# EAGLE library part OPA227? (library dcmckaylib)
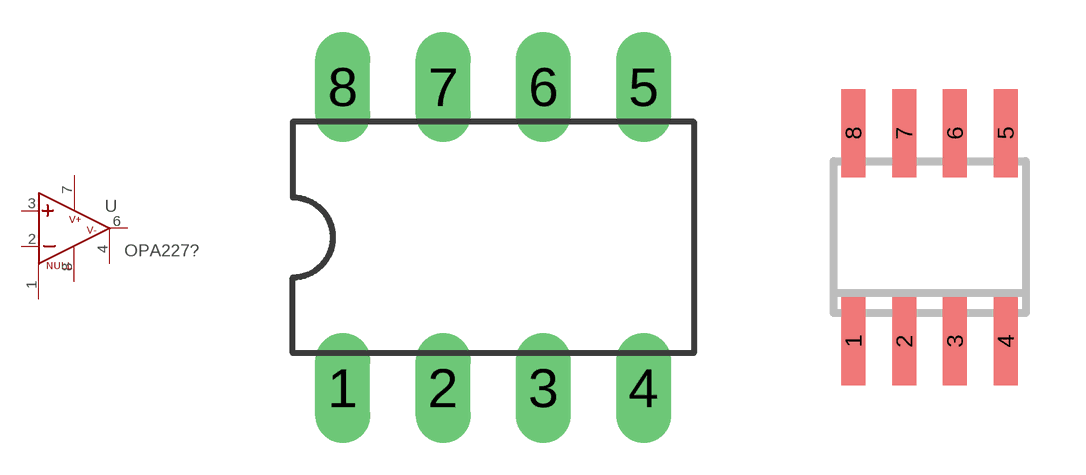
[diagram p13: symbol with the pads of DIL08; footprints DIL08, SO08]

Designator prefix U

## OPA227P  [DIL08]
1  NULL1
2  IN-  in
3  IN+  in
4  V-  pwr
6  OUT  out
7  V+  pwr
8  NULL2

## OPA227U  [SO08]
Pads as for DIL08

## Footprint DIL08 (pad centres in mm)
Dual In Line Package
drill 0.889 long: 1 -3.81,-3.81; 2 -1.27,-3.81; 3 1.27,-3.81; 4 3.81,-3.81; 5 3.81,3.81; 6 1.27,3.81; 7 -1.27,3.81; 8 -3.81,3.81

## Footprint SO08 (pad centres in mm)
Small Outline Package 8 NS Package M08A
smd 0.6 x 2.2: 1 -1.905,-2.6; 2 -0.635,-2.6; 3 0.635,-2.6; 4 1.905,-2.6; 5 1.905,2.6; 6 0.635,2.6; 7 -0.635,2.6; 8 -1.905,2.6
